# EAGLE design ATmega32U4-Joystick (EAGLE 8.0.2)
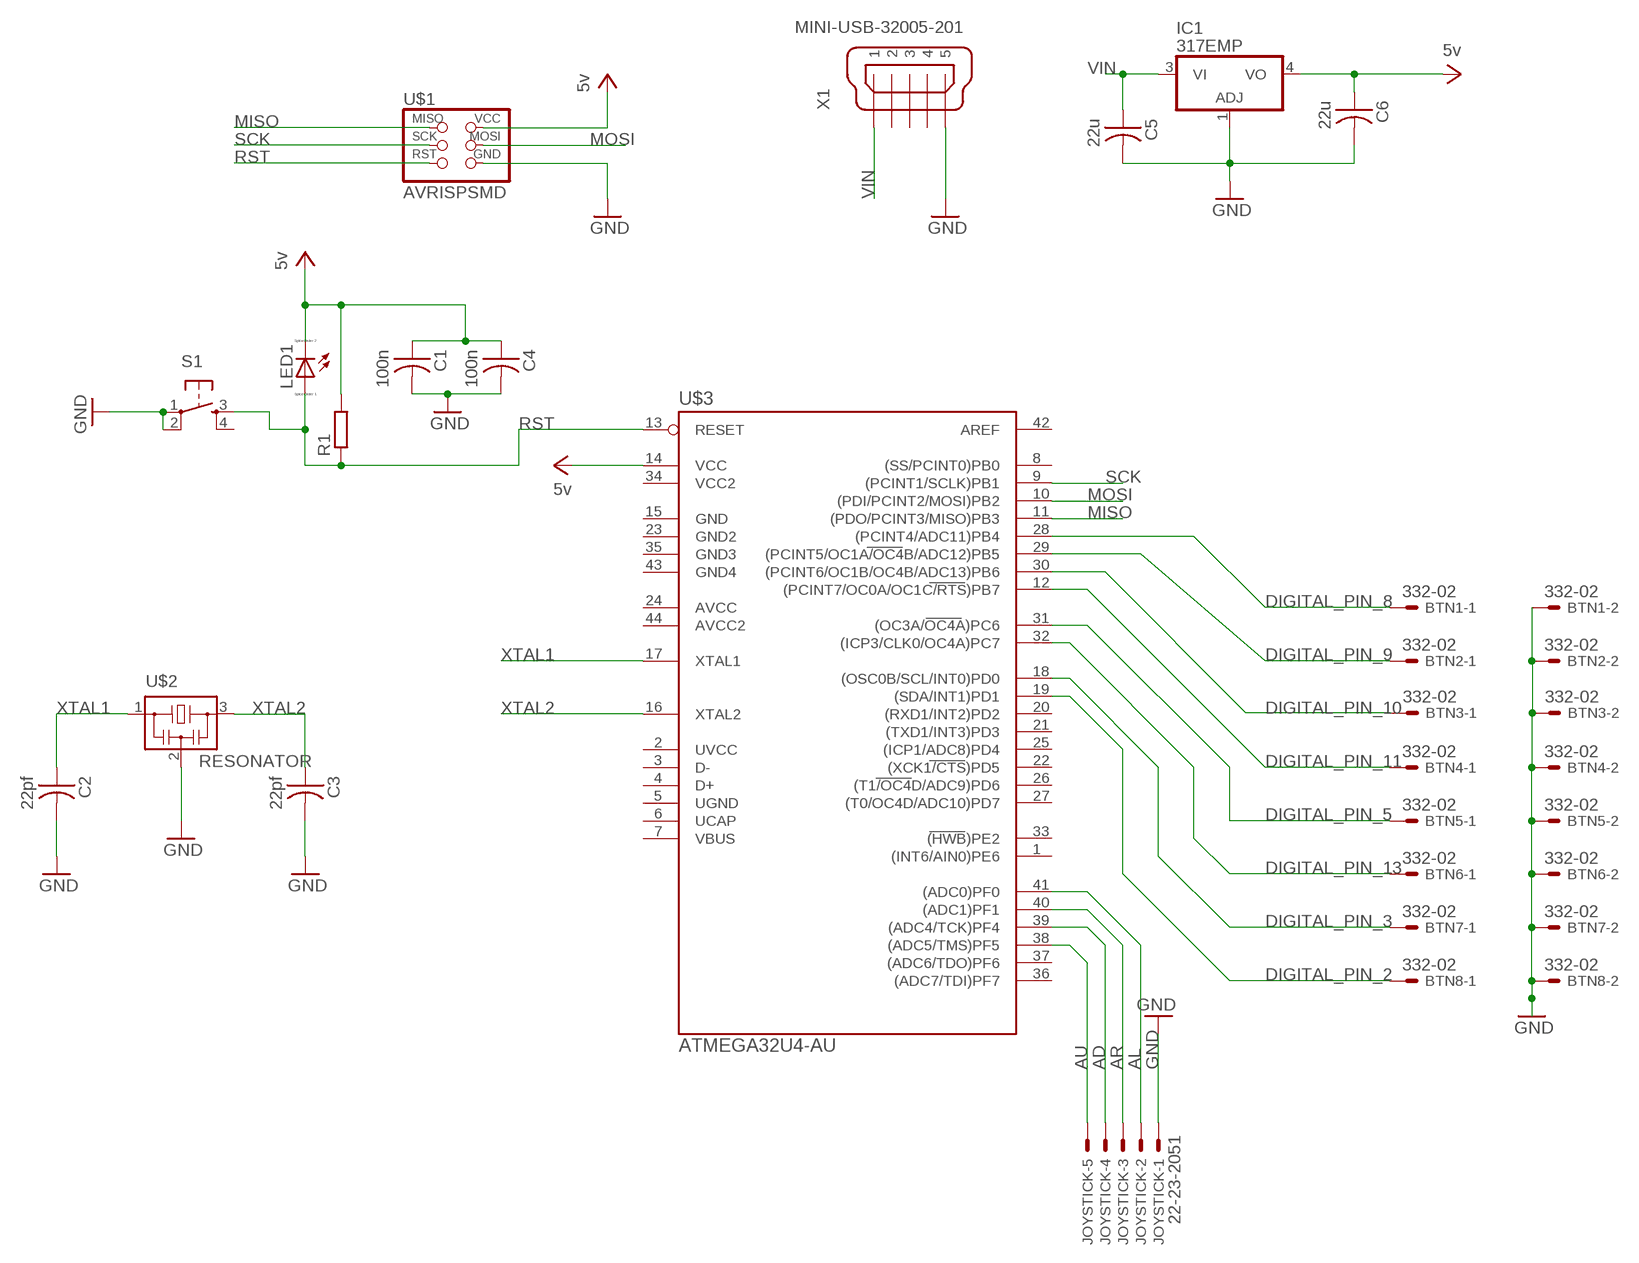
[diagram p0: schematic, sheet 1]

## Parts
BTN1  332-02  [332-02]
BTN2  332-02  [332-02]
BTN3  332-02  [332-02]
BTN4  332-02  [332-02]
BTN5  332-02  [332-02]
BTN6  332-02  [332-02]
BTN7  332-02  [332-02]
BTN8  332-02  [332-02]
C1  100n  CAP-US1206FAB  [C1206FAB]
C2  22pf  CAP-US1206FAB  [C1206FAB]
C3  22pf  CAP-US1206FAB  [C1206FAB]
C4  100n  CAP-US1206FAB  [C1206FAB]
C5  22u  CAP-US1206FAB  [C1206FAB]
C6  22u  CAP-US1206FAB  [C1206FAB]
IC1  317EMP  [SOT223]
JOYSTICK  22-23-2051  [22-23-2051]
LED1  LED_E  [LED_1206]
R1  R-EU_M0805  [M0805]
S1  6MM_SWITCH6MM_SWITCH  [6MM_SWITCH]
U$1  AVRISPSMD  [2X03SMD]
U$2  RESONATOR  [EFOBM]
U$3  ATMEGA32U4-AU  [TQFP44]
X1  MINI-USB-32005-201  [32005-201]

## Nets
AD: JOYSTICK.4 U$3.39((ADC4/TCK)PF4)
AL: JOYSTICK.2 U$3.41((ADC0)PF0)
AR: JOYSTICK.3 U$3.40((ADC1)PF1)
AU: JOYSTICK.5 U$3.38((ADC5/TMS)PF5)
DIGITAL_PIN_2: BTN8.1 U$3.19((SDA/INT1)PD1)
DIGITAL_PIN_3: BTN7.1 U$3.18((OSC0B/SCL/INT0)PD0)
DIGITAL_PIN_5: BTN5.1 U$3.31((OC3A/OC4A)PC6)
DIGITAL_PIN_8: BTN1.1 U$3.28((PCINT4/ADC11)PB4)
DIGITAL_PIN_9: BTN2.1 U$3.29((PCINT5/OC1A/OC4B/ADC12)PB5)
DIGITAL_PIN_10: BTN3.1 U$3.30((PCINT6/OC1B/OC4B/ADC13)PB6)
DIGITAL_PIN_11: BTN4.1 U$3.12((PCINT7/OC0A/OC1C/RTS)PB7)
DIGITAL_PIN_13: BTN6.1 U$3.32((ICP3/CLK0/OC4A)PC7)
GND: BTN1.2 BTN2.2 BTN3.2 BTN4.2 BTN5.2 BTN6.2 BTN7.2 BTN8.2 C1.2 C2.2 C3.2 C4.2 C5.2 C6.2 IC1.1(ADJ) JOYSTICK.1 S1.1(P) S1.2(P1) U$1.6(GND) U$2.2 X1.5
MISO: U$1.1(MISO) U$3.11((PDO/PCINT3/MISO)PB3)
MOSI: U$1.4(MOSI) U$3.10((PDI/PCINT2/MOSI)PB2)
RST: LED1.A R1.1 S1.3(S) U$1.5(RST) U$3.13(RESET)
SCK: U$1.3(SCK) U$3.9((PCINT1/SCLK)PB1)
VCC: C1.1 C4.1 C6.1 IC1.4(VO) LED1.C R1.2 U$1.2(VCC) U$3.14(VCC) ; supply symbol labelled 5v
VIN: C5.1 IC1.3(VI) X1.1
XTAL1: C2.1 U$2.1 U$3.17(XTAL1)
XTAL2: C3.1 U$2.3 U$3.16(XTAL2)
Unconnected: S1.4(S1) U$3.1((INT6/AIN0)PE6) U$3.2(UVCC) U$3.3(D-) U$3.4(D+) U$3.5(UGND) U$3.6(UCAP) U$3.7(VBUS) U$3.8((SS/PCINT0)PB0) U$3.15(GND) U$3.20((RXD1/INT2)PD2) U$3.21((TXD1/INT3)PD3) U$3.22((XCK1/CTS)PD5) U$3.23(GND2) U$3.24(AVCC) U$3.25((ICP1/ADC8)PD4) U$3.26((T1/OC4D/ADC9)PD6) U$3.27((T0/OC4D/ADC10)PD7) U$3.33((HWB)PE2) U$3.34(VCC2) U$3.35(GND3) U$3.36((ADC7/TDI)PF7) U$3.37((ADC6/TDO)PF6) U$3.42(AREF) U$3.43(GND4) U$3.44(AVCC2) X1.2 X1.3 X1.4

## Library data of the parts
BTN1-BTN8 = con-garry:332-02: 2 Pin - 2mm Dual Row
C1-C6 = fab:CAP-US
IC1 = linear:*317: Positive VOLTAGE REGULATOR
JOYSTICK = con-molex:22-23-2051: .100" (2.54mm) Center Header - 5 Pin; MF: MOLEX; MPN: 22-23-2051; OC_FARNELL: 1462952; OC_NEWARK: 38C9178
LED1 = eagle-ltspice:LED_E: LED; SPICEMODEL: NONE; SPICEPREFIX: D; SPICETYPE: diode
R1 = resistor:R-EU_: RESISTOR, European symbol
S1 = fab:6MM_SWITCH: OMRON SWITCH
U$1 = fab:AVRISP
U$2 = fab:RESONATOR
U$3 = mega32U4:ATMEGA32U4-AU
X1 = con-cypressindustries:MINI-USB-: MINI USB-B Conector Source: www.cypressindustries.com; OC_FARNELL: unknown; OC_NEWARK: unknown

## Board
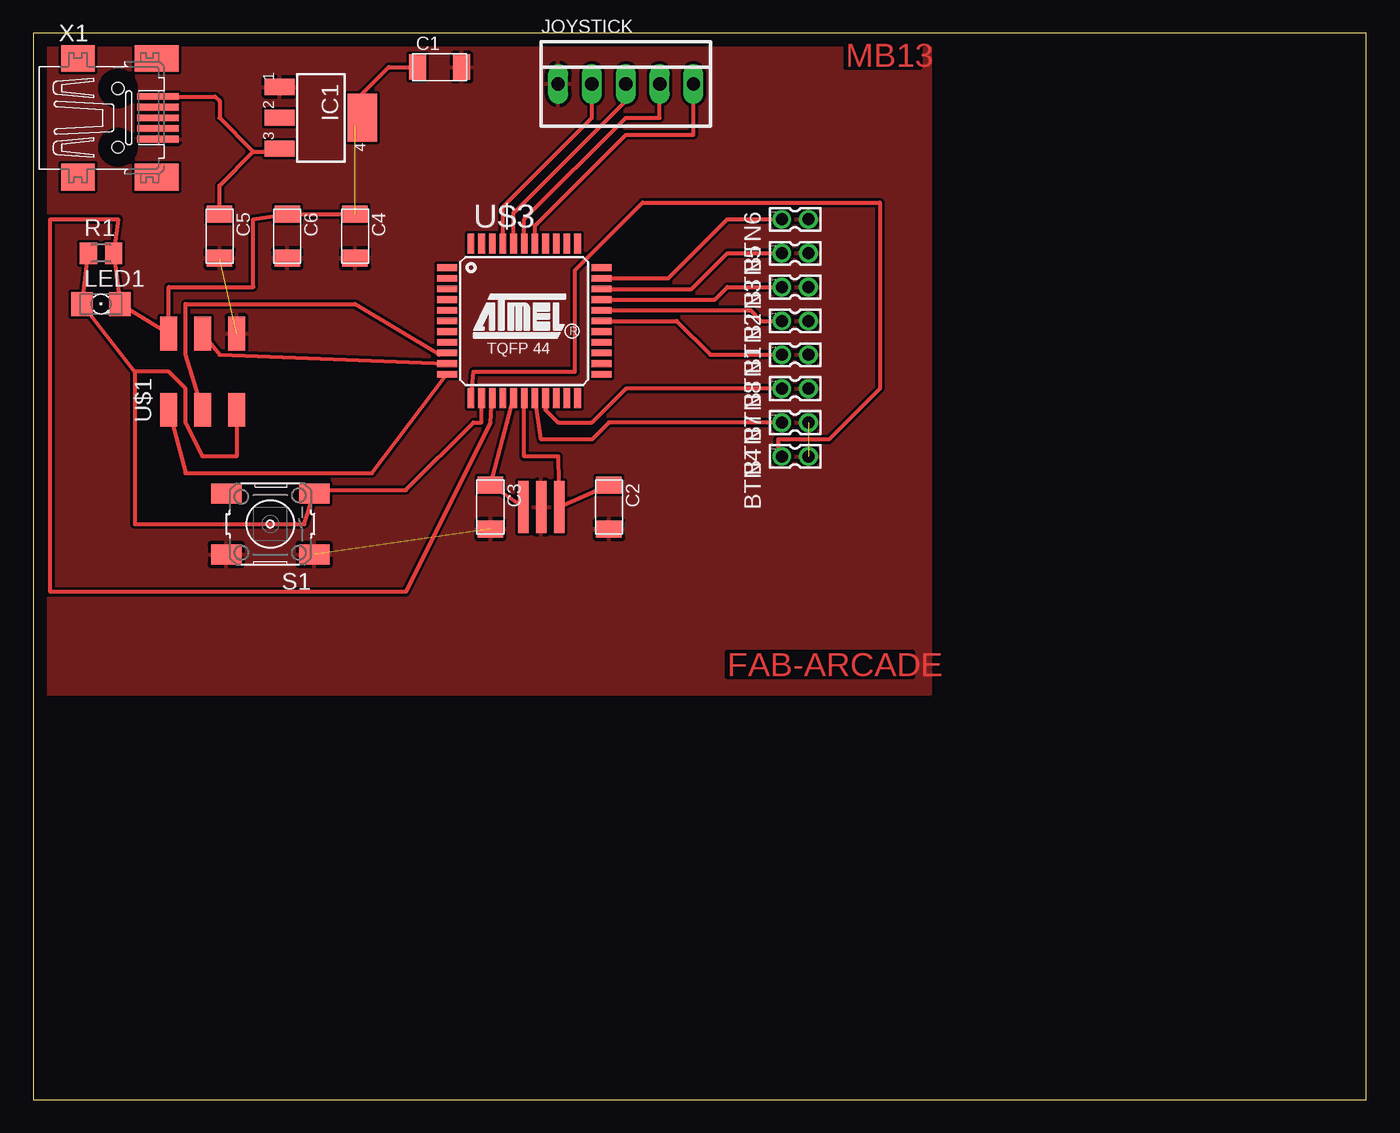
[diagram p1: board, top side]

Size 100 x 80 mm. Coordinates in mm from the lower left corner, seen from the top.
Outline: 0,0 100,0 100,80 0,80 0,0
Copper layers (1*16): Top 0.035mm / dielectric 1.5mm / Bottom 0.035mm
Design rules "default": minimum track width 10mil, minimum drill 24mil, track to track 8mil, track to pad 8mil, pad to pad 8mil, via to via 8mil, smd to smd 8mil, copper to edge 40mil, drill to drill 8mil, minimum pad ring 10mil, minimum via ring 8mil, stop-mask expansion 4mil, vias tented up to drill 0mil, thermal gap 10mil

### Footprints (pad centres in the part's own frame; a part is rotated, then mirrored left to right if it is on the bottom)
332-02 = drill 0.9 pad 1.27: 1 0,-1; 2 0,1
C1206FAB = smd 1.27 x 1.905: 1 -1.651,0; 2 1.651,0
SOT223 = smd 1.219 x 2.235: 1 -2.311,-3.099; 2 0,-3.099; 3 2.311,-3.099 | smd 3.6 x 2.2: 4 0,3.099
22-23-2051 = drill 1 long: 1 -5.08,0; 2 -2.54,0; 3 0,0; 4 2.54,0; 5 5.08,0
LED_1206 = smd 1.6 x 1.803: A -1.422,0; C 1.422,0
M0805 = smd 1.3 x 1.6: 1 -0.95,0; 2 0.95,0
6MM_SWITCH = smd 2.286 x 1.524: 1 -3.302,2.286; 2 3.302,2.286; 3 -3.302,-2.286; 4 3.302,-2.286
2X03SMD = smd 2.54 x 1.27: 1 -2.857,2.54; 2 2.857,2.54; 3 -2.857,0; 4 2.857,0; 5 -2.857,-2.54; 6 2.857,-2.54
EFOBM = smd 0.8 x 3.9: 1 -1.35,0; 2 0,0; 3 1.35,0
TQFP44 = smd 1.5 x 0.5: 1 -5.8,4; 2 -5.8,3.2; 3 -5.8,2.4; 4 -5.8,1.6; 5 -5.8,0.8; 6 -5.8,0; 7 -5.8,-0.8; 8 -5.8,-1.6; 9 -5.8,-2.4; 10 -5.8,-3.2; 11 -5.8,-4; 23 5.8,-4; 24 5.8,-3.2; 25 5.8,-2.4; 26 5.8,-1.6; 27 5.8,-0.8; 28 5.8,0; 29 5.8,0.8; 30 5.8,1.6; 31 5.8,2.4; 32 5.8,3.2; 33 5.8,4 | smd 0.5 x 1.5: 12 -4,-5.8; 13 -3.2,-5.8; 14 -2.4,-5.8; 15 -1.6,-5.8; 16 -0.8,-5.8; 17 0,-5.8; 18 0.8,-5.8; 19 1.6,-5.8; 20 2.4,-5.8; 21 3.2,-5.8; 22 4,-5.8; 34 4,5.8; 35 3.2,5.8; 36 2.4,5.8; 37 1.6,5.8; 38 0.8,5.8; 39 0,5.8; 40 -0.8,5.8; 41 -1.6,5.8; 42 -2.4,5.8; 43 -3.2,5.8; 44 -4,5.8
32005-201 = smd 3.1 x 0.5: 1 3,1.6; 2 3,0.8; 3 3,0; 4 3,-0.8; 5 3,-1.6 | smd 2.5 x 2: M1 -3,-4.45; M2 -3,4.45 | smd 3.3 x 2: M3 2.9,4.45; M4 2.9,-4.45 | hole 0.9: 0,2.2; 0,-2.2

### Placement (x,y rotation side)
BTN1  57.15,55.88 270 top
BTN2  57.15,58.42 270 top
BTN3  57.15,60.96 270 top
BTN4  57.15,48.26 270 top
BTN5  57.15,63.5 270 top
BTN6  57.15,66.04 270 top
BTN7  57.15,50.8 270 top
BTN8  57.15,53.34 270 top
C1  30.48,77.47 0 top
C2  43.18,44.45 270 top
C3  34.29,44.45 270 top
C4  24.13,64.77 270 top
C5  13.97,64.77 270 top
C6  19.05,64.77 270 top
IC1  21.59,73.66 270 top
JOYSTICK  44.45,76.2 0 top
LED1  5.08,59.69 0 top
R1  5.08,63.5 0 top
S1  17.78,43.18 180 top
U$1  12.7,54.61 90 top
U$2  38.1,44.45 180 top
U$3  36.83,58.42 0 top
X1  6.35,73.66 0 top

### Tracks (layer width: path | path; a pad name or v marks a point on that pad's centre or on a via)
AD
  Top 0.305: U$3.39 36.83,66.04 44.45,73.66 46.99,73.66 JOYSTICK.4
AL
  Top 0.305: U$3.41 35.23,66.98 41.91,73.66 JOYSTICK.2
AR
  Top 0.305: U$3.40 36.03,66.51 44.45,74.93 JOYSTICK.3
AU
  Top 0.305: U$3.38 37.63,65.57 44.45,72.39 49.53,72.39 JOYSTICK.5
DIGITAL_PIN_2
  Top 0.305: BTN8.1 44.45,53.34 41.91,50.8 39.37,50.8 38.43,51.74 U$3.19
DIGITAL_PIN_3
  Top 0.305: BTN7.1 43.18,50.8 41.91,49.53 38.1,49.53 U$3.18
DIGITAL_PIN_5
  Top 0.305: U$3.31 49.39,60.82 52.07,63.5 BTN5.1
DIGITAL_PIN_8
  Top 0.305: U$3.28 48.26,58.42 50.8,55.88 BTN1.1
DIGITAL_PIN_9
  Top 0.305: U$3.29 53.81,59.22 54.61,58.42 BTN2.1
DIGITAL_PIN_10
  Top 0.305: U$3.30 51.13,60.02 52.07,60.96 BTN3.1
DIGITAL_PIN_11
  Top 0.305: BTN4.1 55.88,48.53 55.88,49.53 59.69,49.53 63.5,53.34 63.5,67.31 45.72,67.31 40.64,62.23 40.64,54.61 33.02,54.61 U$3.12
DIGITAL_PIN_13
  Top 0.305: U$3.32 47.65,61.62 52.07,66.04 BTN6.1
GND  (3 unrouted)
  pour Top: 0,30.48 67.31,30.48 67.31,31.75 67.31,80.01 0,80.01 0,78.74
MISO
  Top 0.305: U$1.1 11.43,46.99 25.4,46.99 U$3.11
MOSI
  Top 0.305: U$1.4 13.97,55.88 U$3.10
RST
  Top 0.305: U$3.13 33.63,50.8 33.02,50.8 27.94,45.72 21.34,45.72 S1.3 20.32,43.18 7.62,43.18 7.62,54.61 | U$1.5 15.24,48.26 12.7,48.26 11.43,50.8 11.43,53.34 10.16,54.61 7.62,54.61 | 7.62,54.61 LED1.A R1.1
SCK
  Top 0.305: U$1.3 11.43,55.88 11.43,59.69 24.13,59.69 30.48,55.88 U$3.9
VCC  (1 unrouted)
  Top 0.305: C1.1 26.67,77.47 24.69,75.49 IC1.4 24.13,73.1 | C4.1 C6.1 16.51,66.04 16.51,60.96 10.16,60.96 U$1.2 LED1.C R1.2 6.35,66.04 1.27,66.04 1.27,38.1 27.94,38.1 34.29,50.8 U$3.14
VIN
  Top 0.305: X1.1 13.64,75.26 13.97,74.93 13.97,73.66 16.51,71.12 | 16.51,71.12 18.26,71.12 IC1.3 | C5.1 13.97,68.58 16.51,71.12
XTAL1
  Top 0.305: 36.91,52.54 U$3.17 36.83,48.26 39.37,48.26 U$2.1 C2.1
XTAL2
  Top 0.305: U$3.16 35.56,50.8 C3.1 U$2.3

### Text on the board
Top: MB13 | FAB-ARCADE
